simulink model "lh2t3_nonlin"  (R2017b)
settings: Solver=ode45  StartTime=0.0  StopTime=10.0  RelTol=1e-3  EnableMultiTasking=on
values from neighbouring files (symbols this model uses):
  amp = 1.8    [lh2t3.m]
  k = 1    [lh2t3.m]
  L = 1    [lh2t3.m]
  R = 1    [lh2t3.m]
  u0 = 4    [lh2t3.m]

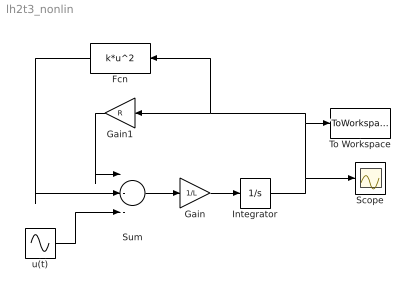
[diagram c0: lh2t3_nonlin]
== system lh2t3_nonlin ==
  Fcn : Fcn  Expr=k*u^2
  Gain : Gain  Gain=1/L
  Gain1 : Gain  Gain=R
  Integrator : Integrator  InitialCondition=-R/(2*k)+sqrt(R^2/(4*k^2)+u0/k)
  Scope : Scope
  Sum : Sum  Inputs=|--+
  To Workspace : ToWorkspace  VariableName=i_nonlin  SampleTime=-1
  u(t) : Sin  Amplitude=amp  Bias=u0  SampleTime=0
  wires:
  u(t)/1 -> Sum/3
  Integrator/1 -> Scope/1, Gain1/1, Fcn/1, To Workspace/1
  Gain1/1 -> Sum/1
  Fcn/1 -> Sum/2
  Sum/1 -> Gain/1
  Gain/1 -> Integrator/1
